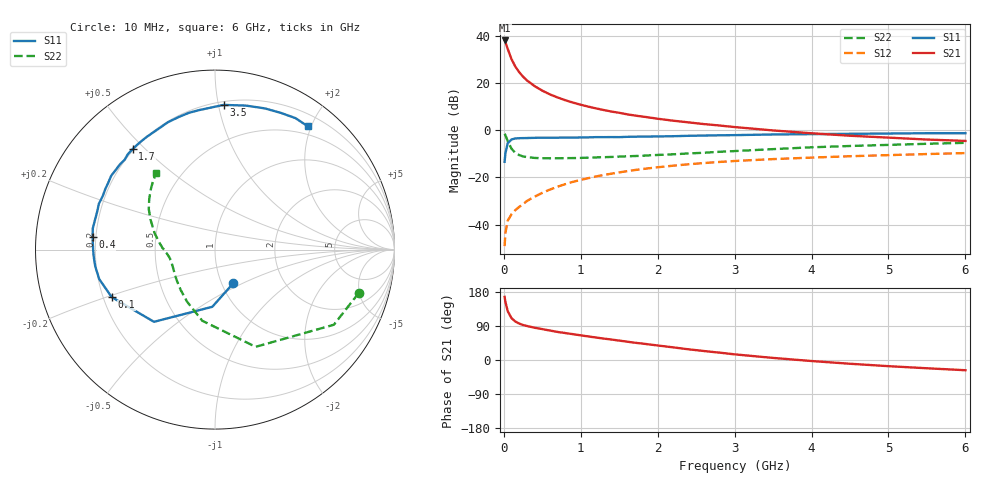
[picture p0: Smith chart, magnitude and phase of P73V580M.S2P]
! SIEMENS Small Signal Semiconductors
! BFP196
! Si NPN RF Bipolar Junction Transistor in SOT143
! VCE = 3.5 V  IC = 80 mA
! Common Emitter S-Parameters:  May  1996
# GHz  S  MA  R  50
!  f  S11  S21  S12  S22
! GHz  MAG  ANG  MAG  ANG  MAG  ANG  MAG  ANG
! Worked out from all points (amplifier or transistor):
!   36 points, 10 MHz to 6 GHz, reference 50 ohm
!   highest |S21| = 37.9 dB at 10 MHz (marker M1)
!   |S21| within 3 dB of that: start of sweep to 44.24 MHz
!   unconditionally stable (mu >= 1): 365 MHz to 4.722 GHz
!   at 250 MHz: K = 0.92, MSG = 27.0 dB, |S12| = -31.3 dB
!   at 1.4 GHz: K = 1.09, MAG = 11.3 dB, |S12| = -18.4 dB
!   at 6 GHz: K = 0.98, MSG = 2.6 dB, |S12| = -9.7 dB
!   S11 on the Smith chart (normalised r, x): 10 MHz: 1.13, -0.45; 100 MHz: 0.23, -0.21; 400 MHz: 0.19, +0.05; 1.7 GHz: 0.19, +0.46; 3.5 GHz: 0.22, +1.04; 6 GHz: 0.37, +1.95
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0.01  0.2134 -61.4  78.76 166.7  0.0035 76.7  0.8366 -16.8
0.02  0.319 -92.7  72.72 153.8  0.0066 66.6  0.7835 -32.3
0.05  0.5267 -130.2  52.35 129.1  0.0121 55.5  0.5872 -67.3
0.1  0.6335 -155.3  31.6 110.3  0.0166 51.7  0.4028 -100.1
0.15  0.6656 -165.7  21.98 101.4  0.0203 52.6  0.329 -118.3
0.2  0.6738 -172.0  16.78 96.1  0.0237 57.0  0.2955 -130.2
0.25  0.6771 -176.8  13.46 92.3  0.0271 59.7  0.2772 -138.9
0.3  0.679 -180.0  11.26 89.7  0.0316 61.7  0.2682 -144.5
0.4  0.6858 174.1  8.516 85.2  0.039 64.1  0.2577 -152.8
0.5  0.691 170.1  6.823 81.5  0.047 65.4  0.2536 -158.4
0.6  0.6887 165.9  5.687 77.7  0.0552 65.6  0.2531 -161.9
0.7  0.69 161.7  4.894 74.0  0.0636 65.2  0.2535 -164.6
0.9  0.693 154.4  3.81 68.1  0.0805 63.7  0.2558 -168.9
1.1  0.7019 147.9  3.129 62.1  0.0963 61.8  0.2611 -171.9
1.3  0.7091 141.3  2.653 56.5  0.1123 59.1  0.267 -174.6
1.7  0.7246 129.3  2.035 45.7  0.1425 53.4  0.2824 -179.7
2.2  0.742 115.6  1.58 33.4  0.1766 45.6  0.3075 174.1
3  0.7822 96.5  1.159 14.9  0.2219 33.5  0.3596 162.2
3.5  0.8076 86.6  0.983 5.5  0.2434 26.4  0.3958 155.1
4.5  0.8344 70.5  0.759 -9.9  0.2799 14.2  0.4609 142.7
5.5  0.8589 58.5  0.631 -21.8  0.3112 3.5  0.5129 132.5
6  0.8598 53.0  0.59 -27.0  0.3262 -2.2  0.5375 127.6
